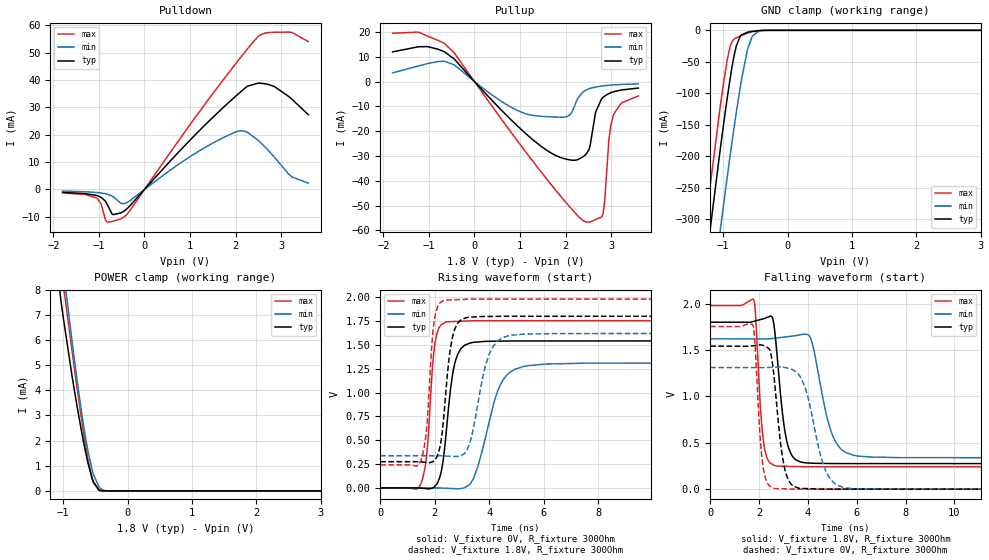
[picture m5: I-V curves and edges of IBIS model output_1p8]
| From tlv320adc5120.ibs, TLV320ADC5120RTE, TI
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|   output_1p8 Model
[Model]   output_1p8
Model_type   3-state
Polarity   Non-Inverting
Vmeas = 0.9
Vref = 0
Cref = 2pF
Rref = 100000
|   typ   min   max
C_comp   2.727pF   2.727pF   2.778pF
| Where Nom  PVT is Nominal Process, 1.8V, 27C
|   Fast PVT is Strong Process,  1.98V, -40C
|   Slow PVT is Weak Process,   1.62V, 150C
[Voltage Range]   1.8   1.62   1.98
|Junction Temperature
[Temperature Range]   27   150   -40
[Pullup Reference]   1.8   1.62   1.98
[Pulldown Reference]   0   0   0
[Power Clamp Reference]   1.8   1.62   1.98
[GND Clamp Reference]   0   0   0
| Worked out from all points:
|   slope of the pulldown table from 0 to 0.27 V, typ, clamps not added: 54.1 ohm
|   slope of the pullup table from 0 to 0.27 V, typ, clamps not added: 50.4 ohm
|   GND clamp passes 1 mA (typ) near -0.50 V on its own axis
|   POWER clamp passes 1 mA (typ) near -0.60 V on its own axis
|   falling waveform, V_fixture 1.8V, R_fixture 300Ohm: 20-80 % time 369ps typ, 644ps min, 240ps max; typ from 1.8 V to 0.275 V
|   rising waveform, V_fixture 0V, R_fixture 300Ohm: 20-80 % time 365ps typ, 739ps min, 254ps max; typ from 0 V to 1.54 V
|   rising waveform, V_fixture 1.8V, R_fixture 300Ohm: 20-80 % time 323ps typ, 558ps min, 244ps max; typ from 0.275 V to 1.8 V
|   falling waveform, V_fixture 0V, R_fixture 300Ohm: 20-80 % time 381ps typ, 700ps min, 242ps max; typ from 1.54 V to 0 V
[Pulldown]
|   Voltage   I(typ)   I(min)   I(max)
-1.8V     -1.069mA   -586.5uA   -1.279mA
-1.06V    -2.172mA   -1.1mA     -3.078mA
-957.6mV  -2.829mA   -1.289mA   -5.128mA
-817.2mV  -5.528mA   -1.724mA   -11.97mA
-687.6mV  -9.216mA   -2.605mA   -11.62mA
-444.6mV  -7.876mA   -5.197mA   -10mA
1.348V    23.88mA    15.51mA    31.61mA
2.018V    34.3mA     21.12mA    46.28mA
2.266V    37.79mA    20.85mA    51.49mA
2.714V    38.43mA    14.38mA    57.37mA
3.211V    33.4mA     4.999mA    57.48mA
3.6V      27.33mA    2.289mA    54.08mA
[GND Clamp]
|   Voltage   I(typ)   I(min)   I(max)
-1.8V     -840mA     -962.7mA   -775.7mA
-1.46V    -537.9mA   -664.7mA   -470.8mA
-1.222V   -333.5mA   -462.7mA   -264.6mA
-1.195V   -310.9mA   -440.2mA   -241.9mA
-1.055V   -196.6mA   -325.6mA   -128.4mA
-1.006V   -158.8mA   -287mA     -92.29mA
-930.6mV  -103.2mA   -228.4mA   -43.62mA
-822.6mV  -36.7mA    -149.1mA   -13.45mA
-714.6mV  -7.165mA   -78.29mA   -8.153mA
-547.2mV  -1.562mA   -9.154mA   -2.368mA
-433.8mV  -329uA     -867.4uA   -578.4uA
3.6V      0A         0A         0A
[Pullup]
|   Voltage   I(typ)   I(min)   I(max)
-1.8V     11.96mA    3.513mA    19.47mA
-1.033V   14.1mA     7.233mA    18.32mA
-444.6mV  9.09mA     6.732mA    11.59mA
1.273V    -23.29mA   -13.61mA   -31.89mA
2.034V    -31.35mA   -14.11mA   -49.24mA
2.444V    -29.44mA   -3.47mA    -56.54mA
2.542V    -25.73mA   -2.746mA   -56.6mA
2.66V     -12.37mA   -2.203mA   -55.62mA
2.822V    -6.404mA   -1.748mA   -53.34mA
2.952V    -4.839mA   -1.505mA   -23.61mA
3.065V    -4.069mA   -1.346mA   -12.93mA
3.6V      -2.623mA   -919uA     -5.795mA
[POWER Clamp]
|   Voltage   I(typ)   I(min)   I(max)
-1.8V     26.52mA    27.36mA    28.31mA
-1.157V   10.19mA    12.35mA    11.12mA
-1.033V   7.548mA    9.587mA    8.876mA
-1.006V   7.032mA    8.998mA    8.37mA
-860.4mV  4.547mA    5.92mA     5.546mA
-714.6mV  2.37mA     3.14mA     2.846mA
-612mV    1.084mA    1.55mA     1.228mA
-531mV    359.5uA    667uA      333.5uA
-444.6mV  40.63uA    167.5uA    19.38uA
-374.4mV  3.381uA    34.59uA    698.2nA
-261mV    9.783nA    1.563uA    0A
3.6V      0A         0A         0A
[Ramp]
R_load = 300
|   typ   min   max
dV/dt_r   0.924893/3.64639e-10   0.786564/7.37288e-10   1.05212/2.53001e-10
dV/dt_f   0.915033/3.67724e-10   0.769123/6.41731e-10   1.04315/2.39848e-10
[Falling Waveform]
V_fixture = 1.8V
V_fixture_min = 1.62V
V_fixture_max = 1.98V
R_fixture = 300Ohm
C_fixture = 0F
|   Time   V(typ)   V(min)   V(max)
0s        1.8V       1.62V      1.98V
1.788ns   1.81V      1.619V     2.036V
2.172ns   1.837V     1.619V     529.2mV
2.646ns   1.689V     1.627V     253mV
3.097ns   563.8mV    1.642V     246.4mV
3.659ns   296.3mV    1.662V     242.9mV
4.123ns   280.2mV    1.619V     241.7mV
5.027ns   276mV      567.5mV    241.7mV
5.864ns   275.7mV    365.7mV    241.7mV
20ns      274.9mV    338.1mV    241.4mV
[Rising Waveform]
V_fixture = 0V
V_fixture_min = 0V
V_fixture_max = 0V
R_fixture = 300Ohm
C_fixture = 0F
|   Time   V(typ)   V(min)   V(max)
0s        2.068nV    -291.2nV   1.229nV
1.492ns   -1.109mV   85.57uV    43mV
1.711ns   -7.604mV   98.21uV    366.4mV
2.007ns   19.1mV     115.2uV    1.514V
2.41ns    551.9mV    -3.192mV   1.739V
2.67ns    1.215V     -6.541mV   1.744V
2.97ns    1.464V     -5.436mV   1.748V
4.441ns   1.539V     1.1V       1.753V
5.266ns   1.541V     1.274V     1.753V
20ns      1.541V     1.311V     1.754V
[Rising Waveform]
V_fixture = 1.8V
V_fixture_min = 1.62V
V_fixture_max = 1.98V
R_fixture = 300Ohm
C_fixture = 0F
|   Time   V(typ)   V(min)   V(max)
0s        274.9mV    338.1mV    241.4mV
1.487ns   273.9mV    338.2mV    284.6mV
1.698ns   267mV      338.2mV    612.9mV
1.975ns   288.5mV    338.2mV    1.741V
2.325ns   725.3mV    335.8mV    1.965V
2.816ns   1.715V     330.1mV    1.974V
3.299ns   1.79V      483.5mV    1.979V
4.011ns   1.798V     1.409V     1.98V
4.712ns   1.8V       1.596V     1.98V
20ns      1.8V       1.62V      1.98V
[Falling Waveform]
|Gnd
V_fixture = 0V
V_fixture_min = 0V
V_fixture_max = 0V
R_fixture = 300Ohm
C_fixture = 0F
|   Time   V(typ)   V(min)   V(max)
0s        1.541V     1.311V     1.754V
1.751ns   1.546V     1.31V      1.766V
2.131ns   1.551V     1.31V      300.3mV
2.573ns   1.304V     1.314V     11.59mV
3.024ns   247.3mV    1.314V     3.744mV
3.575ns   13.4mV     1.25V      298.8uV
3.977ns   5.874mV    1.015V     291.4uV
4.712ns   434.1uV    208.9mV    278.1uV
5.421ns   413.9uV    21.15mV    265.2uV
20ns      2.066nV    -291.7nV   1.204nV
